DATA_BLOCK "DB_WARNING"
TITLE =
{ S7_language := '9(1) Inglese (Stati Uniti)  09.12.2014  12:08:08' }
VERSION : 0.1


  STRUCT
   D25_Q01 : BOOL ;	//S.T. CONDIZIONATORE
   D25_F01 : BOOL ;	//TEMPERATURA ALTA ARMADIO ELETTRICO
   E54_Q01 : BOOL ;	//S.T. GRU ORIENTABILE
   E54_XY28_0 : BOOL ;	//GRU ORIENTABILE FUORI POSIZIONE
   E09_S01_HH : BOOL ;	//ALTISSIMO LIVELLO OLIO CENTRALINA IDRAULICA
   E09_S01_H : BOOL ;	//ALTO LIVELLO OLIO CENTRALINA IDRAULICA
   E09_S01_L : BOOL ;	//BASSO LIVELLO OLIO CENTRALINA IDRAULICA
   E09_S01_LL : BOOL ;	//BASSISSIMO LIVELLO OLIO CENTRALINA IDRAULICA
   E51_T01 : BOOL ;	//ALTA CORRENTE MOTORE FRESATRICE PLANETARIA 1
   E52_T01 : BOOL ;	//ALTA CORRENTE MOTORE FRESATRICE PLANETARIA 2
   E61_S11_1 : BOOL ;	//BASSO LIVELLO OLIO LUBRIFICAZIONE 1
   E62_S17_1 : BOOL ;	//BASSO LIVELLO OLIO LUBRIFICAZIONE 2 WG1
   E62_S17_4 : BOOL ;	//BASSO LIVELLO OLIO LUBRIFICAZIONE 2 WG2
   E63_B11_4 : BOOL ;	//BASSO LIVELLO OLIO LUBRIFICAZIONE 3
   E08_S02_3 : BOOL ;	//MANCATA PARTENZA EVACUATORE TRUCIOLI 1
   E08_S28_6 : BOOL ;	//MANCATA PARTENZA EVACUATORE TRUCIOLI 2
   E08_S28_7 : BOOL ;	//MANCATA PARTENZA EVACUATORE TRUCIOLI 3
   E61_S11_11 : BOOL ;	//BASSO LIVELLO OLIO LUBRIFICAZIONE 1
   E61_F20_0 : BOOL ;	//MANCANZA PRESSIONE LUBRIFICAZIONE CONTROPUNTA 1
   E61_F20_1 : BOOL ;	//MANCANZA PRESSIONE LUBRIFICAZIONE GUIDA CONTROPUNTA 1
   E61_F20_2 : BOOL ;	//MANCANZA PRESSIONE LUBRIFICAZIONE SLITTA A CROCE 1
   E61_F20_3 : BOOL ;	//MANCANZA PRESSIONE LUBRIFICAZIONE GUIDA FRESATRICE 1
   E61_F20_4 : BOOL ;	//MANCANZA PRESSIONE LUBRIFICAZIONE FRESATRICE 1
   E61_F21_2 : BOOL ;	//MANCANZA PRESSIONE LUBRIFICAZIONE SERRAGGIO SUPPLEMENTARE 1
   E61_F20_5 : BOOL ;	//MANCANZA PRESSIONE LUBRIFICAZIONE CONTROPUNTA 2
   E61_F20_6 : BOOL ;	//MANCANZA PRESSIONE LUBRIFICAZIONE GUIDA CONTROPUNTA 2
   E61_F20_7 : BOOL ;	//MANCANZA PRESSIONE LUBRIFICAZIONE SLITTA A CROCE 2
   E61_F21_0 : BOOL ;	//MANCANZA PRESSIONE LUBRIFICAZIONE GUIDA FRESATRICE 2
   E61_F21_1 : BOOL ;	//MANCANZA PRESSIONE LUBRIFICAZIONE FRESATRICE 2
   E62_F17_6 : BOOL ;	//INTASAMENTO FILTRO OLIO LUBRIFICAZIONE 2 WG1
   E62_F17_0 : BOOL ;	//MANCANZA PRESSIONE LUBRIFICAZIONE 2 WG1
   E62_S17_1_1 : BOOL ;	//BASSO LIVELLO OLIO LUBRIFICAZIONE 2 WG1
   E62_F17_7 : BOOL ;	//INTASAMENTO FILTRO OLIO LUBRIFICAZIONE 2 WG2
   E62_F17_3 : BOOL ;	//MANCANZA PRESSIONE LUBRIFICAZIONE 2 WG2
   E62_S17_4_1 : BOOL ;	//BASSO LIVELLO OLIO LUBRIFICAZIONE 2 WG2
   E63_B11_41 : BOOL ;	//BASSO LIVELLO OLIO LUBRIFICAZIONE 3
   E63_F21_4 : BOOL ;	//MANCANZA LUBRIFICAZIONE 3 RIDOTTA MONTANTE 1
   E63_F21_5 : BOOL ;	//MANCANZA LUBRIFICAZIONE 3 MONTANTE 1
   E63_F21_6 : BOOL ;	//MANCANZA LUBRIFICAZIONE 3 RIDOTTA MONTANTE 2
   E63_F21_7 : BOOL ;	//MANCANZA LUBRIFICAZIONE 3 MONTANTE 2
   G76_F28_5 : BOOL ;	//MANCANZA PEZZO SU MANDRINO
   E09_F01_3 : BOOL ;	//INTASAMENTO FILTRO OLIO CENTRALINA IDRAULICA
   M01_R01 : BOOL ;	//ALTA TEMPERATURA SU CONTROPUNTA 1
   M02_R01 : BOOL ;	//ALTA TEMPERATURA SU CONTROPUNTA 2
   M05_R01 : BOOL ;	//ALTA TEMPERATURA SU FRESATRICE PLANETARIA 1
   M06_R01 : BOOL ;	//ALTA TEMPERATURA SU FRESATRICE PLANETARIA 2
   M44X21 : BOOL ;	//PORTALE IN INTERFERENZA
   RICETTA_1 : BOOL ;	//TIPO ALBERO DIVERSO DA QUELLO IN MACCHINA
   UTENSILE_1 : BOOL ;	//UTENSILE 1 FINE LAVORAZIONE
   UTENSILE_2 : BOOL ;	//UTENSILE 2 FINE LAVORAZIONE
   FRESE_OFF : BOOL ;	//FRESE FERME
   PORTALE : BOOL ;	//TIME OUT PORTALE
   TEMPO_CICLO : BOOL ;	//TEMPO CICLO MAGGIORE DI QUELLO IMPOSTATO
   PORTALE_CODICE : BOOL ;	//CODICE PEZZO PORTALE INCONGRUENTE
   SPARE14 : BOOL ;
   ALLARME : BOOL ;
   ALLARME1 : BOOL ;	//ASSE Z CONTROPUNTA BLOCCATA E ACCOPPIATA
   ALLARME2 : BOOL ;	//ASSE Z CONTROPUNTA NON BLOCCATA E NON ACCOPPIATA
   ALLARME3 : BOOL ;	//ASSE Z CONTROPUNTA BLOCCATA
   ALLARME4 : BOOL ;	//ASSE Z CONTROPUNTA ACCOPPIATA IN RICERCA DI ZERO
   ALLARME5 : BOOL ;	//ASSE Z SLITTA A CROCE BLOCCATA
   ALLARME6 : BOOL ;	//ASSE Z SLITTA A CROCE NON SBLOCCATA
   ALLARME7 : BOOL ;	//ASSE Z SPORTELLO TRUCIOLI NON APERTO
   ALLARME8 : BOOL ;	//ASSE Z MANCA INTERBLOCCO CON ASSE X
   ALLARME9 : BOOL ;	//ASSE Z MANCA INTERBLOCCO CON ASSE C
   ALLARME10 : BOOL ;
   ALLARME11 : BOOL ;	//ASSE Z2 CONTROPUNTA BLOCCATA E ACCOPPIATA
   ALLARME12 : BOOL ;	//ASSE Z2 CONTROPUNTA NON BLOCCATA E NON ACCOPPIATA
   ALLARME13 : BOOL ;	//ASSE Z2 CONTROPUNTA BLOCCATA
   ALLARME14 : BOOL ;	//ASSE Z2 CONTROPUNTA ACCOPPIATA IN RICERCA DI ZERO
   ALLARME15 : BOOL ;	//ASSE Z2 SLITTA A CROCE BLOCCATA
   ALLARME16 : BOOL ;	//ASSE Z2 SLITTA A CROCE NON SBLOCCATA
   ALLARME17 : BOOL ;	//ASSE Z2 SPORTELLO TRUCIOLI NON APERTO
   ALLARME18 : BOOL ;	//ASSE Z2 MANCA INTERBLOCCO CON ASSE X2
   ALLARME19 : BOOL ;	//ASSE Z2 MANCA INTERBLOCCO CON ASSE C2
   ALLARME20 : BOOL ;	//ASSE X MANCA INTERBLOCCO CON ASSE Z
   ALLARME21 : BOOL ;	//ASSE C MANCA INTERBLOCCO CON ASSE Z
   ALLARME22 : BOOL ;	//ASSE X2 MANCA INTERBLOCCO CON ASSE Z2
   ALLARME23 : BOOL ;	//ASSE C2 MANCA INTERBLOCCO CON ASSE Z2
   ALLARME24 : BOOL ;
   ALLARME25 : BOOL ;
   ALLARME26 : BOOL ;
   ALLARME27 : BOOL ;
   ALLARME28 : BOOL ;
   ALLARME29 : BOOL ;
   ALLARME30 : BOOL ;
   ALLARME31 : BOOL ;
   ALLARME32 : BOOL ;
   ALLARME33 : BOOL ;
   ALLARME34 : BOOL ;
   ALLARME35 : BOOL ;
   ALLARME36 : BOOL ;
   ALLARME37 : BOOL ;
   ALLARME38 : BOOL ;
   ALLARME39 : BOOL ;
   ALLARME40 : BOOL ;
  END_STRUCT ;
BEGIN
   D25_Q01 := FALSE;
   D25_F01 := FALSE;
   E54_Q01 := FALSE;
   E54_XY28_0 := FALSE;
   E09_S01_HH := FALSE;
   E09_S01_H := FALSE;
   E09_S01_L := FALSE;
   E09_S01_LL := FALSE;
   E51_T01 := FALSE;
   E52_T01 := FALSE;
   E61_S11_1 := FALSE;
   E62_S17_1 := FALSE;
   E62_S17_4 := FALSE;
   E63_B11_4 := FALSE;
   E08_S02_3 := FALSE;
   E08_S28_6 := FALSE;
   E08_S28_7 := FALSE;
   E61_S11_11 := FALSE;
   E61_F20_0 := FALSE;
   E61_F20_1 := FALSE;
   E61_F20_2 := FALSE;
   E61_F20_3 := FALSE;
   E61_F20_4 := FALSE;
   E61_F21_2 := FALSE;
   E61_F20_5 := FALSE;
   E61_F20_6 := FALSE;
   E61_F20_7 := FALSE;
   E61_F21_0 := FALSE;
   E61_F21_1 := FALSE;
   E62_F17_6 := FALSE;
   E62_F17_0 := FALSE;
   E62_S17_1_1 := FALSE;
   E62_F17_7 := FALSE;
   E62_F17_3 := FALSE;
   E62_S17_4_1 := FALSE;
   E63_B11_41 := FALSE;
   E63_F21_4 := FALSE;
   E63_F21_5 := FALSE;
   E63_F21_6 := FALSE;
   E63_F21_7 := FALSE;
   G76_F28_5 := FALSE;
   E09_F01_3 := FALSE;
   M01_R01 := FALSE;
   M02_R01 := FALSE;
   M05_R01 := FALSE;
   M06_R01 := FALSE;
   M44X21 := FALSE;
   RICETTA_1 := FALSE;
   UTENSILE_1 := FALSE;
   UTENSILE_2 := FALSE;
   FRESE_OFF := FALSE;
   PORTALE := FALSE;
   TEMPO_CICLO := FALSE;
   PORTALE_CODICE := FALSE;
   SPARE14 := FALSE;
   ALLARME := FALSE;
   ALLARME1 := FALSE;
   ALLARME2 := FALSE;
   ALLARME3 := FALSE;
   ALLARME4 := FALSE;
   ALLARME5 := FALSE;
   ALLARME6 := FALSE;
   ALLARME7 := FALSE;
   ALLARME8 := FALSE;
   ALLARME9 := FALSE;
   ALLARME10 := FALSE;
   ALLARME11 := FALSE;
   ALLARME12 := FALSE;
   ALLARME13 := FALSE;
   ALLARME14 := FALSE;
   ALLARME15 := FALSE;
   ALLARME16 := FALSE;
   ALLARME17 := FALSE;
   ALLARME18 := FALSE;
   ALLARME19 := FALSE;
   ALLARME20 := FALSE;
   ALLARME21 := FALSE;
   ALLARME22 := FALSE;
   ALLARME23 := FALSE;
   ALLARME24 := FALSE;
   ALLARME25 := FALSE;
   ALLARME26 := FALSE;
   ALLARME27 := FALSE;
   ALLARME28 := FALSE;
   ALLARME29 := FALSE;
   ALLARME30 := FALSE;
   ALLARME31 := FALSE;
   ALLARME32 := FALSE;
   ALLARME33 := FALSE;
   ALLARME34 := FALSE;
   ALLARME35 := FALSE;
   ALLARME36 := FALSE;
   ALLARME37 := FALSE;
   ALLARME38 := FALSE;
   ALLARME39 := FALSE;
   ALLARME40 := FALSE;
END_DATA_BLOCK

